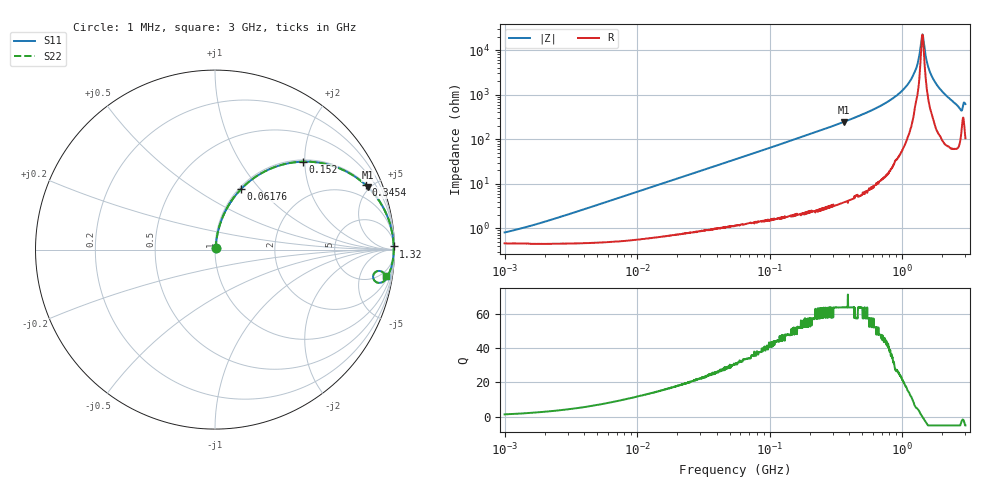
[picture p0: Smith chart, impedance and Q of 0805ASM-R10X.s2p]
!s-Parameter Generated by FASTRON Sdn. Bhd.
!FASTRON P/N : 0805ASM-R10X
!Keysight Technologies: E4991B_MY54100416_A.01.15
!Date: Fri Jun 19 14:50:04 2026
!Version  :Rev00  Fri Jun 19 14:50:04 2026
!Data & Calibration Information:
!Freq  S11  S21  S12  S22
!PortZ  Port1:50+j0  Port2:50+j0
!When reading reference impedance value at option line is always used.
! Remarks : This data is being provided solely for informational purposes.
# Hz S dB R 50
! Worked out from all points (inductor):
!   1601 points, 1 MHz to 3 GHz, reference 50 ohm
!   read as one part in series: L = 106 nH near 2.025 MHz
!   highest Q = 63.7 at 363.1 MHz (marker M1), where L = 107 nH
!   self-resonance near 1.423 GHz
!   S11 on the Smith chart (normalised r, x): 1 MHz: 1.01, +0.01; 61.76 MHz: 1.02, +0.79; 152 MHz: 1.04, +1.95; 345.4 MHz: 1.08, +4.63; 1.32 GHz: open; 3 GHz: 3, -12
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1000000  -41.80 54.9  -0.04 -0.4  -0.04 -0.4  -41.80 54.9
3804036  -31.80 78.1  -0.04 -1.4  -0.04 -1.4  -31.80 78.1
1.447069e7  -20.50 80.8  -0.09 -5.4  -0.09 -5.4  -20.50 80.8
5.504702e7  -9.61 68.8  -0.60 -19.3  -0.60 -19.3  -9.61 68.8
6.176144e7  -8.75 66.8  -0.73 -21.4  -0.73 -21.4  -8.75 66.8
1.520175e8  -3.20 45.1  -2.99 -43.8  -2.99 -43.8  -3.20 45.1
2.083556e8  -1.98 36.2  -4.57 -52.8  -4.57 -52.8  -1.98 36.2
3.453811e8  -0.79 23.2  -8.08 -65.9  -8.08 -65.9  -0.79 23.2
3.631036e8  -0.72 22.1  -8.49 -67.0  -8.49 -67.0  -0.72 22.1
7.925923e8  -0.11 7.9  -17.20 -80.7  -17.20 -80.7  -0.11 7.9
9.538021e8  -0.07 5.3  -20.70 -82.4  -20.70 -82.4  -0.07 5.3
1.113852e9  -0.05 3.2  -25.00 -82.9  -25.00 -82.9  -0.05 3.2
1.243477e9  -0.04 1.7  -30.20 -79.6  -30.20 -79.6  -0.04 1.7
1.320433e9  -0.04 1.0  -34.90 -75.6  -34.90 -75.6  -0.04 1.0
1.388188e9  -0.04 0.3  -43.10 -51.0  -43.10 -51.0  -0.04 0.3
1.430499e9  -0.04 -0.1  -46.80 13.5  -46.80 13.5  -0.04 -0.1
1.45942e9  -0.04 -0.3  -42.90 52.2  -42.90 52.2  -0.04 -0.3
1.534307e9  -0.04 -1.0  -34.80 74.9  -34.80 74.9  -0.04 -1.0
1.596974e9  -0.04 -1.6  -31.20 78.5  -31.20 78.5  -0.04 -1.6
1.818868e9  -0.06 -3.4  -24.60 81.2  -24.60 81.2  -0.06 -3.4
2.714296e9  -0.44 -11.0  -14.30 69.8  -14.30 69.8  -0.44 -11.0
3e9  -0.34 -8.8  -16.10 71.3  -16.10 71.3  -0.34 -8.8
